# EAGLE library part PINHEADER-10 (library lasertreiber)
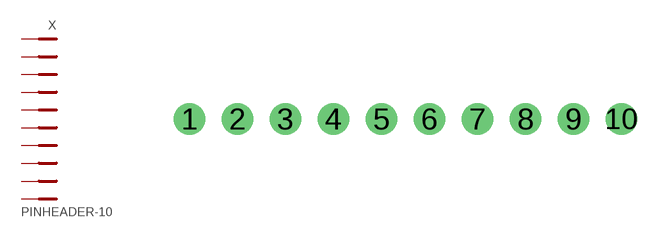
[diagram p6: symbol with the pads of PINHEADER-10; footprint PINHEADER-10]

Designator prefix X

## PINHEADER-10  [PINHEADER-10]
1  1
2  2
3  3
4  4
5  5
6  6
7  7
8  8
9  9
10  10

## Footprint PINHEADER-10 (pad centres in mm)
drill 1.1: 1 -11.43,0; 2 -8.89,0; 3 -6.35,0; 4 -3.81,0; 5 -1.27,0; 6 1.27,0; 7 3.81,0; 8 6.35,0; 9 8.89,0; 10 11.43,0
